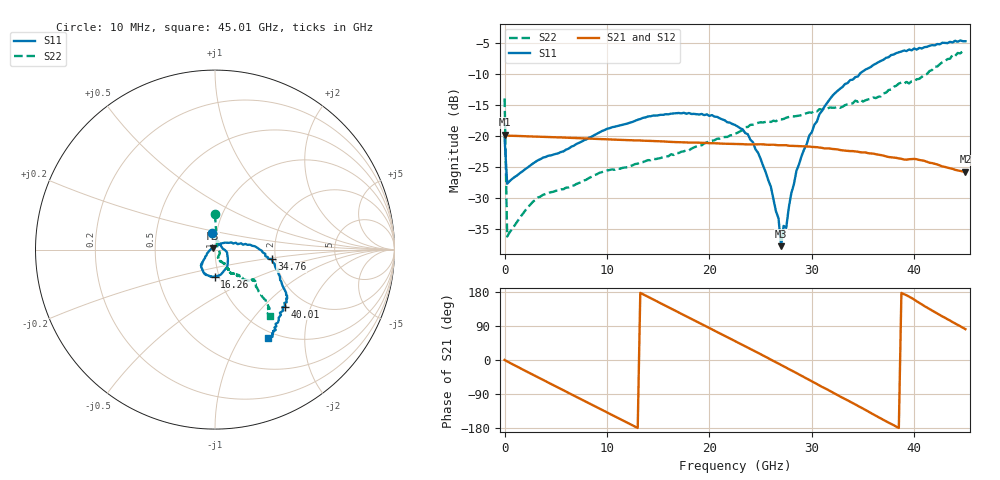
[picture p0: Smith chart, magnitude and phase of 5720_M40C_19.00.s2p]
! Device:  ADRF5720
! Description: 0.5dB LSB GaAs MMIC 6-bit Digital Attenuator
! Frequency:  0.000009 -  40 GHz
! Ports:
!	RF1	= Port 1
!	RF2	= Port 2
! Vdd:  3.3 Volt
! Vss:  -3.3 Volt
! Control:  0/3.3 Volt
! State:  19.00 dB attenuation
! Data:  The device was measured using G-S-G Probes on a matrix board.
!  Data was collected using an calibrated 4 port network analyzer.
!  The reference plane for this measurement is at the launchers.
! Note:  Analog Devices supplies this data as a sample of measured data
!  for this product.  Your particular data for this product may vary.
!  Data was taken at -40 degrees C.
!  Analog Devices reserves the right to change this data at anytime.
# GHZ S DB R 45.0
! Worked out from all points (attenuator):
!   181 points, 10 MHz to 45.01 GHz, reference 45 ohm
!   highest |S21| = -19.81 dB at 10 MHz (marker M1); lowest = -25.8 dB at 45.01 GHz (marker M2)
!   lowest |S11| = -37.8 dB at 27.01 GHz (marker M3), VSWR 1.03, Z = 44.1 + j0.691 ohm
!   |S11| at or under -10 dB: start of sweep to 34.72 GHz
!   |S22| runs from -36.2 to -6.3 dB; largest |S21 - S12| = 0.00045
!   S11 on the Smith chart (normalised r, x): 10 MHz: 0.95, +0.18; 16.26 GHz: 0.95, -0.29; 34.76 GHz: 1.90, -0.23; 40.01 GHz: 1.58, -1.35; 45.01 GHz: 0.90, -1.34
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0.01  -20.40 98.6  -19.81 0.2  -19.83 0.2  -13.98 90.2
0.26  -27.75 13.0  -19.99 -3.8  -20.01 -3.8  -36.25 32.1
3.26  -23.96 -8.8  -20.16 -45.6  -20.18 -45.6  -29.96 -32.0
7.76  -20.73 -38.6  -20.43 -107.5  -20.45 -107.5  -27.23 -65.4
15.26  -16.63 -84.2  -20.90 149.5  -20.92 149.4  -23.59 -68.2
16.26  -16.45 -90.5  -21.00 135.7  -21.02 135.7  -22.99 -66.3
20.26  -16.68 -114.1  -21.21 80.8  -21.23 80.7  -20.83 -57.9
22.76  -18.51 -131.5  -21.34 46.5  -21.37 46.5  -19.53 -58.0
24.26  -21.04 -137.0  -21.40 26.0  -21.42 25.9  -18.23 -56.8
25.51  -25.89 -152.8  -21.44 8.0  -21.46 7.9  -17.77 -55.7
26.76  -33.31 160.0  -21.54 -9.5  -21.55 -9.7  -17.38 -55.4
27.01  -37.80 142.5  -21.53 -12.9  -21.55 -13.0  -17.39 -57.0
27.26  -34.53 118.7  -21.53 -16.6  -21.56 -16.7  -17.30 -55.4
27.51  -34.86 74.6  -21.53 -20.3  -21.55 -20.4  -17.10 -56.7
28.01  -29.26 50.4  -21.63 -27.2  -21.65 -27.3  -16.87 -57.2
28.51  -25.66 42.5  -21.66 -34.4  -21.68 -34.5  -16.83 -56.9
30.26  -18.23 18.0  -21.82 -59.7  -21.85 -59.8  -15.98 -56.5
32.01  -13.59 5.8  -22.13 -85.0  -22.15 -85.1  -15.49 -53.1
34.76  -9.90 -9.6  -22.67 -124.7  -22.69 -124.8  -14.19 -49.2
37.76  -7.00 -29.8  -23.48 -168.7  -23.51 -168.8  -12.55 -45.4
40.01  -5.94 -39.0  -23.74 159.4  -23.76 159.2  -11.19 -39.0
45.01  -4.77 -59.0  -25.82 81.4  -25.86 81.3  -6.33 -50.6
